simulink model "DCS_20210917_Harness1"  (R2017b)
settings: Solver=FixedStepDiscrete  StartTime=0.0  StopTime=10.0  FixedStep=0.01  RelTol=1e-3  EnableMultiTasking=on
undefined symbols (not defined in the file): sigbuilder_block
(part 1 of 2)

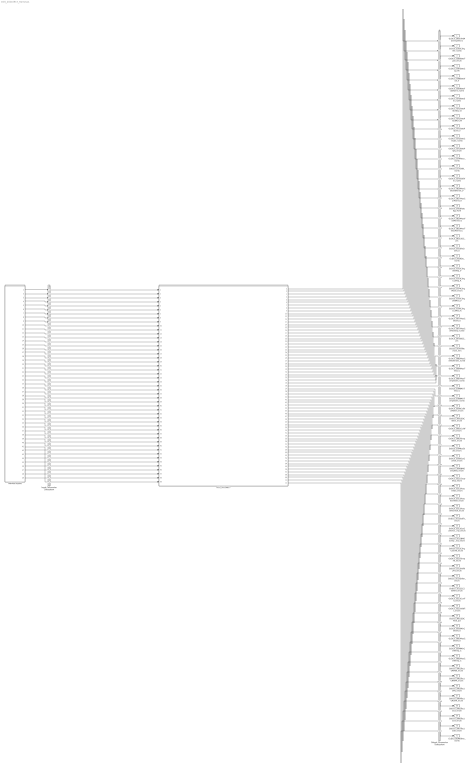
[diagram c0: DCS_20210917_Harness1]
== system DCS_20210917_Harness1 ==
  DCS_20210917 : ModelReference  ModelNameDialog=DCS_20210917  SimulationMode=Normal  ModelReferenceVersion='M106C105'
  Harness Inputs : Subsystem  Tag=STV Subsys  LoadFcn=sigbuilder_block('load');  StartFcn=sigbuilder_block('start');  StopFcn=sigbuilder_block('stop');  ClipboardFcn=sigbuilder_block('clipboard');  mask(Sigbuilder block){tuvar=[0:10]}
      mask init:
      | if ~strcmp(get_param(bdroot(gcb),'SimulationStatus'),'stopped'),tuvar = sigbuilder_block('maskInit'); end
  Input Conversion Subsystem : Subsystem  Tag=__SLT_ICS__  Description=Signal spec. and routing
  Output Conversion Subsystem : Subsystem  Tag=__SLT_OCS__  Description=Signal spec. and routing
  GcDCS_2601AlwMaxChrgVolt_V : Outport  OutDataTypeStr=fixdt('ufix16_Sp1')  PortDimensions=[1]
  GcDCS_2565ChrgVer_numb : Outport  Port=2  OutDataTypeStr=uint32  PortDimensions=[1]
  GeDCS_2566BattType_enum : Outport  Port=3  OutDataTypeStr=uint8  PortDimensions=[1]
  GcDCS_2567BattCap_Ah : Outport  Port=4  OutDataTypeStr=fixdt('ufix16_Sp1')  PortDimensions=[1]
  GcDCS_2568BattVolt_V : Outport  Port=5  OutDataTypeStr=fixdt('ufix16_Sp1')  PortDimensions=[1]
  GaDCS_2569BattFctyName_numb : Outport  Port=6  OutDataTypeStr=uint8  PortDimensions=[4]
  GcDCS_2570BattSer_numb : Outport  Port=7  OutDataTypeStr=uint32  PortDimensions=[1]
  GcDCS_2571BattPrdctDay_D : Outport  Port=8  OutDataTypeStr=uint8  PortDimensions=[1]
  GcDCS_2571BattPrdctMon_M : Outport  Port=9  OutDataTypeStr=uint8  PortDimensions=[1]
  GcDCS_2571BattPrdctYr_Y : Outport  Port=10  OutDataTypeStr=fixdt('ufix8_B1985')  PortDimensions=[1]
  GcDCS_2572BattChrgCt_numb : Outport  Port=11  OutDataTypeStr=uint32  PortDimensions=[1]
  GeDCS_2573BattPrpty_enum : Outport  Port=12  OutDataTypeStr=uint8  PortDimensions=[1]
  GcDCS_2574Resv_numb : Outport  Port=13  OutDataTypeStr=uint8  PortDimensions=[1]
  GaDCS_2575VIN_numb : Outport  Port=14  OutDataTypeStr=uint8  PortDimensions=[17]
  GaDCS_2576SoftVer_numb : Outport  Port=15  OutDataTypeStr=uint8  PortDimensions=[8]
  GcDCS_2816MaxCellVoltPermit_V : Outport  Port=16  OutDataTypeStr=single  PortDimensions=[1]
  GcDCS_2817MaxCurPermit_A : Outport  Port=17  OutDataTypeStr=fixdt('ufix16_Sp1_Bn400')  PortDimensions=[1]
  GcDCS_2818RateEgy_Kwh : Outport  Port=18  OutDataTypeStr=fixdt('ufix16_Sp1')  PortDimensions=[1]
  GcDCS_2819MaxVoltPermit_V : Outport  Port=19  OutDataTypeStr=fixdt('ufix16_Sp1')  PortDimensions=[1]
  GcDCS_2820MaxTempPermit_C : Outport  Port=20  OutDataTypeStr=fixdt('ufix8_Bn50')  PortDimensions=[1]
  GcDCS_2821SOC_pct : Outport  Port=21  OutDataTypeStr=fixdt('ufix16_Sp1')  PortDimensions=[1]
  GcDCS_2822PackVolt_V : Outport  Port=22  OutDataTypeStr=fixdt('ufix16_Sp1')  PortDimensions=[1]
  GcDCS_2829Da_numb : Outport  Port=23  OutDataTypeStr=uint8  PortDimensions=[1]
  GcDCS_3072ChrgVoltReq_V : Outport  Port=24  OutDataTypeStr=fixdt('ufix16_Sp1')  PortDimensions=[1]
  GcDCS_3073ChrgCurReq_A : Outport  Port=25  OutDataTypeStr=fixdt('ufix16_Sp1_Bn400')  PortDimensions=[1]
  GeDCS_3074ChrgMode_enum : Outport  Port=26  OutDataTypeStr=uint8  PortDimensions=[1]
  GcDCS_3075ChrgVoltMea_V : Outport  Port=27  OutDataTypeStr=fixdt('ufix16_Sp1')  PortDimensions=[1]
  GcDCS_3076ChrgCurMea_A : Outport  Port=28  OutDataTypeStr=fixdt('ufix16_Sp1_Bn400')  PortDimensions=[1]
  GcDCS_3077MaxCellVolt_V : Outport  Port=29  OutDataTypeStr=fixdt('ufix16_Sp01')  PortDimensions=[1]
  GcDCS_3077MaxCellVoltGrp_numb : Outport  Port=30  OutDataTypeStr=uint8  PortDimensions=[1]
  GcDCS_3078SOC_pct : Outport  Port=31  OutDataTypeStr=uint8  PortDimensions=[1]
  GcDCS_3079TiRemain_min : Outport  Port=32  OutDataTypeStr=uint16  PortDimensions=[1]
  GcDCS_3085MaxCellVoltIndex_numb : Outport  Port=33  OutDataTypeStr=fixdt('ufix8_B1')  PortDimensions=[1]
  GcDCS_3086MaxTemp_C : Outport  Port=34  OutDataTypeStr=fixdt('ufix8_Bn50')  PortDimensions=[1]
  GcDCS_3087MaxTempIndex_numb : Outport  Port=35  OutDataTypeStr=fixdt('ufix8_B1')  PortDimensions=[1]
  GcDCS_3088MinTemp_C : Outport  Port=36  OutDataTypeStr=fixdt('ufix8_Bn50')  PortDimensions=[1]
  GcDCS_3089MinTempIndex_numb : Outport  Port=37  OutDataTypeStr=fixdt('ufix8_B1')  PortDimensions=[1]
  GeDCS_3090CellVoltWarn_enum : Outport  Port=38  OutDataTypeStr=uint8  PortDimensions=[1]
  GeDCS_3091SOCWarn_enum : Outport  Port=39  OutDataTypeStr=uint8  PortDimensions=[1]
  GeDCS_3092CurWarn_enum : Outport  Port=40  OutDataTypeStr=uint8  PortDimensions=[1]
  GeDCS_3093TempWarn_enum : Outport  Port=41  OutDataTypeStr=uint8  PortDimensions=[1]
  GeDCS_3094IsoState_enum : Outport  Port=42  OutDataTypeStr=uint8  PortDimensions=[1]
  GeDCS_3095OutContSt_enum : Outport  Port=43  OutDataTypeStr=uint8  PortDimensions=[1]
  GeDCS_3096BMSChrgRdy_enum : Outport  Port=44  OutDataTypeStr=uint8  PortDimensions=[1]
  GeDCS_3511ChrgrStop_enum : Outport  Port=45  OutDataTypeStr=uint8  PortDimensions=[1]
  GeDCS_3511ReachSOC_enum : Outport  Port=46  OutDataTypeStr=uint8  PortDimensions=[1]
  GeDCS_3511ReachCellVolt_enum : Outport  Port=47  OutDataTypeStr=uint8  PortDimensions=[1]
  GeDCS_3511ReachPackVolt_enum : Outport  Port=48  OutDataTypeStr=uint8  PortDimensions=[1]
  GeDCS_3512IsoFlt_enum : Outport  Port=49  OutDataTypeStr=uint8  PortDimensions=[1]
  GeDCS_3512OutContOverTemp_enum : Outport  Port=50  OutDataTypeStr=uint8  PortDimensions=[1]
  GeDCS_3512BMSCompOverTemp_enum : Outport  Port=51  OutDataTypeStr=uint8  PortDimensions=[1]
  GeDCS_3512ChrgContFlt_enum : Outport  Port=52  OutDataTypeStr=uint8  PortDimensions=[1]
  GeDCS_3512TempFlt_enum : Outport  Port=53  OutDataTypeStr=uint8  PortDimensions=[1]
  GeDCS_3512HVRlyFlt_enum : Outport  Port=54  OutDataTypeStr=uint8  PortDimensions=[1]
  GeDCS_3512Other_enum : Outport  Port=55  OutDataTypeStr=uint8  PortDimensions=[1]
  GeDCS_3512CC2VoltFlt_enum : Outport  Port=56  OutDataTypeStr=uint8  PortDimensions=[1]
  GeDCS_3513CurrFlt_enum : Outport  Port=57  OutDataTypeStr=uint8  PortDimensions=[1]
  GeDCS_3513VoltFlt_enum : Outport  Port=58  OutDataTypeStr=uint8  PortDimensions=[1]
  GcDCS_3601SOCFinal_pct : Outport  Port=59  OutDataTypeStr=uint8  PortDimensions=[1]
  GcDCS_3602MinCellVolt_V : Outport  Port=60  OutDataTypeStr=fixdt('ufix16_Sp01')  PortDimensions=[1]
  GcDCS_3603MaxCellVolt_V : Outport  Port=61  OutDataTypeStr=fixdt('ufix16_Sp01')  PortDimensions=[1]
  GcDCS_3604MinCellTemp_C : Outport  Port=62  OutDataTypeStr=fixdt('ufix8_Bn50')  PortDimensions=[1]
  GcDCS_3605MaxCellTemp_C : Outport  Port=63  OutDataTypeStr=fixdt('ufix8_Bn50')  PortDimensions=[1]
  GeDCS_3901ToutCRM00_enum : Outport  Port=64  OutDataTypeStr=uint8  PortDimensions=[1]
  GeDCS_3902ToutCRMAA_enum : Outport  Port=65  OutDataTypeStr=uint8  PortDimensions=[1]
  GeDCS_3903ToutCML_enum : Outport  Port=66  OutDataTypeStr=uint8  PortDimensions=[1]
  GeDCS_3904ToutCROAA_enum : Outport  Port=67  OutDataTypeStr=uint8  PortDimensions=[1]
  GeDCS_3905ToutCCS_enum : Outport  Port=68  OutDataTypeStr=uint8  PortDimensions=[1]
  GeDCS_3906ToutCST_enum : Outport  Port=69  OutDataTypeStr=uint8  PortDimensions=[1]
  GeDCS_3907ToutCSD_enum : Outport  Port=70  OutDataTypeStr=uint8  PortDimensions=[1]
  GcDCS_BEMOther_numb : Outport  Port=71  OutDataTypeStr=uint8  PortDimensions=[1]
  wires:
  Harness Inputs/1(GbDCC_BSTMsgCmd_flg) -> Input Conversion Subsystem/1(Inport_1)
  Harness Inputs/2(GcDCC_DCChrgVoltRqst_V) -> Input Conversion Subsystem/2(Inport_2)
  Harness Inputs/3(GbDCC_DCChrgVerSta_flg) -> Input Conversion Subsystem/3(Inport_3)
  Harness Inputs/4(GcDCC_DCChrgCrntRqst_A) -> Input Conversion Subsystem/4(Inport_4)
  Harness Inputs/5(GcHDP_PackCrnt_A) -> Input Conversion Subsystem/5(Inport_5)
  Harness Inputs/6(GcCDP_MaxCellVoltNumb_numb) -> Input Conversion Subsystem/6(Inport_6)
  Harness Inputs/7(GcSOC_DispSOC_pct) -> Input Conversion Subsystem/7(Inport_7)
  Harness Inputs/8(GcDCC_ChrgingTiRem_min) -> Input Conversion Subsystem/8(Inport_8)
  Harness Inputs/9(GcCDP_MaxCellTemp_C) -> Input Conversion Subsystem/9(Inport_9)
  Harness Inputs/10(GcCDP_MaxCellTempNumb_numb) -> Input Conversion Subsystem/10(Inport_10)
  Harness Inputs/11(GcCDP_MinCellTemp_C) -> Input Conversion Subsystem/11(Inport_11)
  Harness Inputs/12(GcCDP_MinCellTempNumb_numb) -> Input Conversion Subsystem/12(Inport_12)
  Harness Inputs/13(GbDCC_DCChrgFinish_flg) -> Input Conversion Subsystem/13(Inport_13)
  Harness Inputs/14(GeISO_ResFltLvl_enum) -> Input Conversion Subsystem/14(Inport_14)
  Harness Inputs/15(GeLDP_DCPlugTempState_enum) -> Input Conversion Subsystem/15(Inport_15)
  Harness Inputs/16(GbISP_TFCellTempHiFltLv2_flg) -> Input Conversion Subsystem/16(Inport_16)
  Harness Inputs/17(GbCTD_DCPosCloseFlt_flg) -> Input Conversion Subsystem/17(Inport_17)
  Harness Inputs/18(GbCTD_DCPosOpenFlt_flg) -> Input Conversion Subsystem/18(Inport_18)
  Harness Inputs/19(GeFTC_FltLevel_enum) -> Input Conversion Subsystem/19(Inport_19)
  Harness Inputs/20(GeSOP_ChrgPwrState_enum) -> Input Conversion Subsystem/20(Inport_20)
  Harness Inputs/21(GbISP_TFCellVoltHiFltLv2_flg) -> Input Conversion Subsystem/21(Inport_21)
  Harness Inputs/22(GcCDP_MinCellVolt_mV) -> Input Conversion Subsystem/22(Inport_22)
  Harness Inputs/23(GcCDP_MaxCellVolt_mV) -> Input Conversion Subsystem/23(Inport_23)
  Harness Inputs/24(GbDCC_CRM00Tout_flg) -> Input Conversion Subsystem/24(Inport_24)
  Harness Inputs/25(GbDCC_CRMAATout_flg) -> Input Conversion Subsystem/25(Inport_25)
  Harness Inputs/26(GbDCC_CMLTout_flg) -> Input Conversion Subsystem/26(Inport_26)
  Harness Inputs/27(GbDCC_CROAATout_flg) -> Input Conversion Subsystem/27(Inport_27)
  Harness Inputs/28(GbDCC_CCSTout_flg) -> Input Conversion Subsystem/28(Inport_28)
  Harness Inputs/29(GbDCC_CSTTout_flg) -> Input Conversion Subsystem/29(Inport_29)
  Harness Inputs/30(GbDCC_CSDTout_flg) -> Input Conversion Subsystem/30(Inport_30)
  Harness Inputs/31(GbGDP_CSTRecOnce_flg) -> Input Conversion Subsystem/31(Inport_31)
  Harness Inputs/32(GcHDP_PackVolt_V) -> Input Conversion Subsystem/32(Inport_32)
  Harness Inputs/33(GeCTC_CtrCtlState_enum) -> Input Conversion Subsystem/33(Inport_33)
  Harness Inputs/34(GbDCC_CROTout_flg) -> Input Conversion Subsystem/34(Inport_34)
  Harness Inputs/35(GbDCC_DCCrntUnctrolFlt_flg) -> Input Conversion Subsystem/35(Inport_35)
  Harness Inputs/36(GbLDP_CC2STG_flg) -> Input Conversion Subsystem/36(Inport_36)
  Harness Inputs/37(GbLDP_CC2VoltRaty_flg) -> Input Conversion Subsystem/37(Inport_37)
  Harness Inputs/38(GcADP_VinCode1_numb) -> Input Conversion Subsystem/38(Inport_38)
  Harness Inputs/39(GcADP_VinCode2_numb) -> Input Conversion Subsystem/39(Inport_39)
  Harness Inputs/40(GcADP_VinCode3_numb) -> Input Conversion Subsystem/40(Inport_40)
  Harness Inputs/41(GcADP_VinCode4_numb) -> Input Conversion Subsystem/41(Inport_41)
  Harness Inputs/42(GcADP_VinCode5_numb) -> Input Conversion Subsystem/42(Inport_42)
  Harness Inputs/43(GcADP_VinCode6_numb) -> Input Conversion Subsystem/43(Inport_43)
  Harness Inputs/44(GcADP_VinCode7_numb) -> Input Conversion Subsystem/44(Inport_44)
  Harness Inputs/45(GcADP_VinCodeNum_numb) -> Input Conversion Subsystem/45(Inport_45)
  Harness Inputs/46(GeCTC_CtrCtlConnMode_enum) -> Input Conversion Subsystem/46(Inport_46)
  Harness Inputs/47(GcUDS_FullChrgCutoffVolt_mV) -> Input Conversion Subsystem/47(Inport_47)
  Harness Inputs/48(GcUDS_BatEnergy_kWh) -> Input Conversion Subsystem/48(Inport_48)
  Harness Inputs/49(GeUDS_CapSel_enum) -> Input Conversion Subsystem/49(Inport_49)
  Output Conversion Subsystem/1(Outport_1) -> GcDCS_2601AlwMaxChrgVolt_V/1
  Output Conversion Subsystem/2(Outport_2) -> GcDCS_2565ChrgVer_numb/1
  Output Conversion Subsystem/3(Outport_3) -> GeDCS_2566BattType_enum/1
  Output Conversion Subsystem/4(Outport_4) -> GcDCS_2567BattCap_Ah/1
  Output Conversion Subsystem/5(Outport_5) -> GcDCS_2568BattVolt_V/1
  Output Conversion Subsystem/6(Outport_6) -> GaDCS_2569BattFctyName_numb/1
  Output Conversion Subsystem/7(Outport_7) -> GcDCS_2570BattSer_numb/1
  Output Conversion Subsystem/8(Outport_8) -> GcDCS_2571BattPrdctDay_D/1
  Output Conversion Subsystem/9(Outport_9) -> GcDCS_2571BattPrdctMon_M/1
  Output Conversion Subsystem/10(Outport_10) -> GcDCS_2571BattPrdctYr_Y/1
  Output Conversion Subsystem/11(Outport_11) -> GcDCS_2572BattChrgCt_numb/1
  Output Conversion Subsystem/12(Outport_12) -> GeDCS_2573BattPrpty_enum/1
  Output Conversion Subsystem/13(Outport_13) -> GcDCS_2574Resv_numb/1
  Output Conversion Subsystem/14(Outport_14) -> GaDCS_2575VIN_numb/1
  Output Conversion Subsystem/15(Outport_15) -> GaDCS_2576SoftVer_numb/1
  Output Conversion Subsystem/16(Outport_16) -> GcDCS_2816MaxCellVoltPermit_V/1
  Output Conversion Subsystem/17(Outport_17) -> GcDCS_2817MaxCurPermit_A/1
  Output Conversion Subsystem/18(Outport_18) -> GcDCS_2818RateEgy_Kwh/1
  Output Conversion Subsystem/19(Outport_19) -> GcDCS_2819MaxVoltPermit_V/1
  Output Conversion Subsystem/20(Outport_20) -> GcDCS_2820MaxTempPermit_C/1
  Output Conversion Subsystem/21(Outport_21) -> GcDCS_2821SOC_pct/1
  Output Conversion Subsystem/22(Outport_22) -> GcDCS_2822PackVolt_V/1
  Output Conversion Subsystem/23(Outport_23) -> GcDCS_2829Da_numb/1
  Output Conversion Subsystem/24(Outport_24) -> GcDCS_3072ChrgVoltReq_V/1
  Output Conversion Subsystem/25(Outport_25) -> GcDCS_3073ChrgCurReq_A/1
  Output Conversion Subsystem/26(Outport_26) -> GeDCS_3074ChrgMode_enum/1
  Output Conversion Subsystem/27(Outport_27) -> GcDCS_3075ChrgVoltMea_V/1
  Output Conversion Subsystem/28(Outport_28) -> GcDCS_3076ChrgCurMea_A/1
  Output Conversion Subsystem/29(Outport_29) -> GcDCS_3077MaxCellVolt_V/1
  Output Conversion Subsystem/30(Outport_30) -> GcDCS_3077MaxCellVoltGrp_numb/1
  Output Conversion Subsystem/31(Outport_31) -> GcDCS_3078SOC_pct/1
  Output Conversion Subsystem/32(Outport_32) -> GcDCS_3079TiRemain_min/1
  Output Conversion Subsystem/33(Outport_33) -> GcDCS_3085MaxCellVoltIndex_numb/1
  Output Conversion Subsystem/34(Outport_34) -> GcDCS_3086MaxTemp_C/1
  Output Conversion Subsystem/35(Outport_35) -> GcDCS_3087MaxTempIndex_numb/1
  Output Conversion Subsystem/36(Outport_36) -> GcDCS_3088MinTemp_C/1
  Output Conversion Subsystem/37(Outport_37) -> GcDCS_3089MinTempIndex_numb/1
  Output Conversion Subsystem/38(Outport_38) -> GeDCS_3090CellVoltWarn_enum/1
  Output Conversion Subsystem/39(Outport_39) -> GeDCS_3091SOCWarn_enum/1
  Output Conversion Subsystem/40(Outport_40) -> GeDCS_3092CurWarn_enum/1
  Output Conversion Subsystem/41(Outport_41) -> GeDCS_3093TempWarn_enum/1
  Output Conversion Subsystem/42(Outport_42) -> GeDCS_3094IsoState_enum/1
  Output Conversion Subsystem/43(Outport_43) -> GeDCS_3095OutContSt_enum/1
  Output Conversion Subsystem/44(Outport_44) -> GeDCS_3096BMSChrgRdy_enum/1
  Output Conversion Subsystem/45(Outport_45) -> GeDCS_3511ChrgrStop_enum/1
  Output Conversion Subsystem/46(Outport_46) -> GeDCS_3511ReachSOC_enum/1
  Output Conversion Subsystem/47(Outport_47) -> GeDCS_3511ReachCellVolt_enum/1
  Output Conversion Subsystem/48(Outport_48) -> GeDCS_3511ReachPackVolt_enum/1
  Output Conversion Subsystem/49(Outport_49) -> GeDCS_3512IsoFlt_enum/1
  Output Conversion Subsystem/50(Outport_50) -> GeDCS_3512OutContOverTemp_enum/1
  Output Conversion Subsystem/51(Outport_51) -> GeDCS_3512BMSCompOverTemp_enum/1
  Output Conversion Subsystem/52(Outport_52) -> GeDCS_3512ChrgContFlt_enum/1
  Output Conversion Subsystem/53(Outport_53) -> GeDCS_3512TempFlt_enum/1
  Output Conversion Subsystem/54(Outport_54) -> GeDCS_3512HVRlyFlt_enum/1
  Output Conversion Subsystem/55(Outport_55) -> GeDCS_3512Other_enum/1
  Output Conversion Subsystem/56(Outport_56) -> GeDCS_3512CC2VoltFlt_enum/1
  Output Conversion Subsystem/57(Outport_57) -> GeDCS_3513CurrFlt_enum/1
  Output Conversion Subsystem/58(Outport_58) -> GeDCS_3513VoltFlt_enum/1
  Output Conversion Subsystem/59(Outport_59) -> GcDCS_3601SOCFinal_pct/1
  Output Conversion Subsystem/60(Outport_60) -> GcDCS_3602MinCellVolt_V/1
  Output Conversion Subsystem/61(Outport_61) -> GcDCS_3603MaxCellVolt_V/1
  Output Conversion Subsystem/62(Outport_62) -> GcDCS_3604MinCellTemp_C/1
  Output Conversion Subsystem/63(Outport_63) -> GcDCS_3605MaxCellTemp_C/1
  Output Conversion Subsystem/64(Outport_64) -> GeDCS_3901ToutCRM00_enum/1
  Output Conversion Subsystem/65(Outport_65) -> GeDCS_3902ToutCRMAA_enum/1
  Output Conversion Subsystem/66(Outport_66) -> GeDCS_3903ToutCML_enum/1
  Output Conversion Subsystem/67(Outport_67) -> GeDCS_3904ToutCROAA_enum/1
  Output Conversion Subsystem/68(Outport_68) -> GeDCS_3905ToutCCS_enum/1
  Output Conversion Subsystem/69(Outport_69) -> GeDCS_3906ToutCST_enum/1
  Output Conversion Subsystem/70(Outport_70) -> GeDCS_3907ToutCSD_enum/1
  Output Conversion Subsystem/71(Outport_71) -> GcDCS_BEMOther_numb/1
  Input Conversion Subsystem/1(Outport_1) -> DCS_20210917/1
  Input Conversion Subsystem/2(Outport_2) -> DCS_20210917/2
  Input Conversion Subsystem/3(Outport_3) -> DCS_20210917/3
  Input Conversion Subsystem/4(Outport_4) -> DCS_20210917/4
  Input Conversion Subsystem/5(Outport_5) -> DCS_20210917/5
  Input Conversion Subsystem/6(Outport_6) -> DCS_20210917/6
  Input Conversion Subsystem/7(Outport_7) -> DCS_20210917/7
  Input Conversion Subsystem/8(Outport_8) -> DCS_20210917/8
  Input Conversion Subsystem/9(Outport_9) -> DCS_20210917/9
  Input Conversion Subsystem/10(Outport_10) -> DCS_20210917/10
  Input Conversion Subsystem/11(Outport_11) -> DCS_20210917/11
  Input Conversion Subsystem/12(Outport_12) -> DCS_20210917/12
  Input Conversion Subsystem/13(Outport_13) -> DCS_20210917/13
  Input Conversion Subsystem/14(Outport_14) -> DCS_20210917/14
  Input Conversion Subsystem/15(Outport_15) -> DCS_20210917/15
  Input Conversion Subsystem/16(Outport_16) -> DCS_20210917/16
  Input Conversion Subsystem/17(Outport_17) -> DCS_20210917/17
  Input Conversion Subsystem/18(Outport_18) -> DCS_20210917/18
  Input Conversion Subsystem/19(Outport_19) -> DCS_20210917/19
  Input Conversion Subsystem/20(Outport_20) -> DCS_20210917/20
  Input Conversion Subsystem/21(Outport_21) -> DCS_20210917/21
  Input Conversion Subsystem/22(Outport_22) -> DCS_20210917/22
  Input Conversion Subsystem/23(Outport_23) -> DCS_20210917/23
  Input Conversion Subsystem/24(Outport_24) -> DCS_20210917/24
  Input Conversion Subsystem/25(Outport_25) -> DCS_20210917/25
  Input Conversion Subsystem/26(Outport_26) -> DCS_20210917/26
  Input Conversion Subsystem/27(Outport_27) -> DCS_20210917/27
  Input Conversion Subsystem/28(Outport_28) -> DCS_20210917/28
  Input Conversion Subsystem/29(Outport_29) -> DCS_20210917/29
  Input Conversion Subsystem/30(Outport_30) -> DCS_20210917/30
  Input Conversion Subsystem/31(Outport_31) -> DCS_20210917/31
  Input Conversion Subsystem/32(Outport_32) -> DCS_20210917/32
  Input Conversion Subsystem/33(Outport_33) -> DCS_20210917/33
  Input Conversion Subsystem/34(Outport_34) -> DCS_20210917/34
  Input Conversion Subsystem/35(Outport_35) -> DCS_20210917/35
  Input Conversion Subsystem/36(Outport_36) -> DCS_20210917/36
  Input Conversion Subsystem/37(Outport_37) -> DCS_20210917/37
  Input Conversion Subsystem/38(Outport_38) -> DCS_20210917/38
  Input Conversion Subsystem/39(Outport_39) -> DCS_20210917/39
  Input Conversion Subsystem/40(Outport_40) -> DCS_20210917/40
  Input Conversion Subsystem/41(Outport_41) -> DCS_20210917/41
  Input Conversion Subsystem/42(Outport_42) -> DCS_20210917/42
  Input Conversion Subsystem/43(Outport_43) -> DCS_20210917/43
  Input Conversion Subsystem/44(Outport_44) -> DCS_20210917/44
  Input Conversion Subsystem/45(Outport_45) -> DCS_20210917/45
  Input Conversion Subsystem/46(Outport_46) -> DCS_20210917/46
  Input Conversion Subsystem/47(Outport_47) -> DCS_20210917/47
  Input Conversion Subsystem/48(Outport_48) -> DCS_20210917/48
  Input Conversion Subsystem/49(Outport_49) -> DCS_20210917/49
  DCS_20210917/1 -> Output Conversion Subsystem/1(Inport_1)
  DCS_20210917/2 -> Output Conversion Subsystem/2(Inport_2)
  DCS_20210917/3 -> Output Conversion Subsystem/3(Inport_3)
  DCS_20210917/4 -> Output Conversion Subsystem/4(Inport_4)
  DCS_20210917/5 -> Output Conversion Subsystem/5(Inport_5)
  DCS_20210917/6 -> Output Conversion Subsystem/6(Inport_6)
  DCS_20210917/7 -> Output Conversion Subsystem/7(Inport_7)
  DCS_20210917/8 -> Output Conversion Subsystem/8(Inport_8)
  DCS_20210917/9 -> Output Conversion Subsystem/9(Inport_9)
  DCS_20210917/10 -> Output Conversion Subsystem/10(Inport_10)
  DCS_20210917/11 -> Output Conversion Subsystem/11(Inport_11)
  DCS_20210917/12 -> Output Conversion Subsystem/12(Inport_12)
  DCS_20210917/13 -> Output Conversion Subsystem/13(Inport_13)
  DCS_20210917/14 -> Output Conversion Subsystem/14(Inport_14)
  DCS_20210917/15 -> Output Conversion Subsystem/15(Inport_15)
  DCS_20210917/16 -> Output Conversion Subsystem/16(Inport_16)
  DCS_20210917/17 -> Output Conversion Subsystem/17(Inport_17)
  DCS_20210917/18 -> Output Conversion Subsystem/18(Inport_18)
  DCS_20210917/19 -> Output Conversion Subsystem/19(Inport_19)
  DCS_20210917/20 -> Output Conversion Subsystem/20(Inport_20)
  DCS_20210917/21 -> Output Conversion Subsystem/21(Inport_21)
  DCS_20210917/22 -> Output Conversion Subsystem/22(Inport_22)
  DCS_20210917/23 -> Output Conversion Subsystem/23(Inport_23)
  DCS_20210917/24 -> Output Conversion Subsystem/24(Inport_24)
  DCS_20210917/25 -> Output Conversion Subsystem/25(Inport_25)
  DCS_20210917/26 -> Output Conversion Subsystem/26(Inport_26)
  DCS_20210917/27 -> Output Conversion Subsystem/27(Inport_27)
  DCS_20210917/28 -> Output Conversion Subsystem/28(Inport_28)
  DCS_20210917/29 -> Output Conversion Subsystem/29(Inport_29)
  DCS_20210917/30 -> Output Conversion Subsystem/30(Inport_30)
  DCS_20210917/31 -> Output Conversion Subsystem/31(Inport_31)
  DCS_20210917/32 -> Output Conversion Subsystem/32(Inport_32)
  DCS_20210917/33 -> Output Conversion Subsystem/33(Inport_33)
  DCS_20210917/34 -> Output Conversion Subsystem/34(Inport_34)
  DCS_20210917/35 -> Output Conversion Subsystem/35(Inport_35)
  DCS_20210917/36 -> Output Conversion Subsystem/36(Inport_36)
  DCS_20210917/37 -> Output Conversion Subsystem/37(Inport_37)
  DCS_20210917/38 -> Output Conversion Subsystem/38(Inport_38)
  DCS_20210917/39 -> Output Conversion Subsystem/39(Inport_39)
  DCS_20210917/40 -> Output Conversion Subsystem/40(Inport_40)
  DCS_20210917/41 -> Output Conversion Subsystem/41(Inport_41)
  DCS_20210917/42 -> Output Conversion Subsystem/42(Inport_42)
  DCS_20210917/43 -> Output Conversion Subsystem/43(Inport_43)
  DCS_20210917/44 -> Output Conversion Subsystem/44(Inport_44)
  DCS_20210917/45 -> Output Conversion Subsystem/45(Inport_45)
  DCS_20210917/46 -> Output Conversion Subsystem/46(Inport_46)
  DCS_20210917/47 -> Output Conversion Subsystem/47(Inport_47)
  DCS_20210917/48 -> Output Conversion Subsystem/48(Inport_48)
  DCS_20210917/49 -> Output Conversion Subsystem/49(Inport_49)
  DCS_20210917/50 -> Output Conversion Subsystem/50(Inport_50)
  DCS_20210917/51 -> Output Conversion Subsystem/51(Inport_51)
  DCS_20210917/52 -> Output Conversion Subsystem/52(Inport_52)
  DCS_20210917/53 -> Output Conversion Subsystem/53(Inport_53)
  DCS_20210917/54 -> Output Conversion Subsystem/54(Inport_54)
  DCS_20210917/55 -> Output Conversion Subsystem/55(Inport_55)
  DCS_20210917/56 -> Output Conversion Subsystem/56(Inport_56)
  DCS_20210917/57 -> Output Conversion Subsystem/57(Inport_57)
  DCS_20210917/58 -> Output Conversion Subsystem/58(Inport_58)
  DCS_20210917/59 -> Output Conversion Subsystem/59(Inport_59)
  DCS_20210917/60 -> Output Conversion Subsystem/60(Inport_60)
  DCS_20210917/61 -> Output Conversion Subsystem/61(Inport_61)
  DCS_20210917/62 -> Output Conversion Subsystem/62(Inport_62)
  DCS_20210917/63 -> Output Conversion Subsystem/63(Inport_63)
  DCS_20210917/64 -> Output Conversion Subsystem/64(Inport_64)
  DCS_20210917/65 -> Output Conversion Subsystem/65(Inport_65)
  DCS_20210917/66 -> Output Conversion Subsystem/66(Inport_66)
  DCS_20210917/67 -> Output Conversion Subsystem/67(Inport_67)
  DCS_20210917/68 -> Output Conversion Subsystem/68(Inport_68)
  DCS_20210917/69 -> Output Conversion Subsystem/69(Inport_69)
  DCS_20210917/70 -> Output Conversion Subsystem/70(Inport_70)
  DCS_20210917/71 -> Output Conversion Subsystem/71(Inport_71)

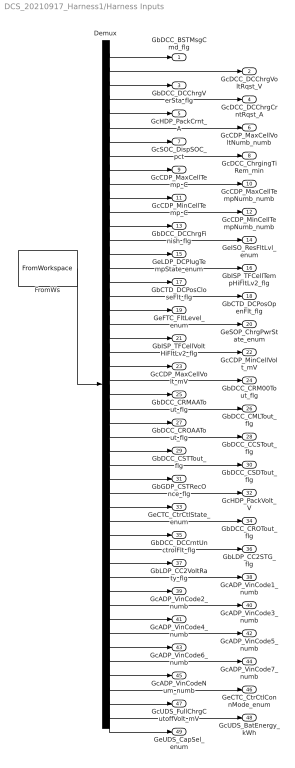
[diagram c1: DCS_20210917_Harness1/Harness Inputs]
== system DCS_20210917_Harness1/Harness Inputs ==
  Demux : Demux  Tag=STV Demux  Outputs=49
  FromWs : FromWorkspace  Tag=STV FromWs  VariableName=tuvar  SampleTime=0
  GbDCC_BSTMsgCmd_flg : Outport  Tag=STV Outport
  GcDCC_DCChrgVoltRqst_V : Outport  Tag=STV Outport  Port=2
  GbDCC_DCChrgVerSta_flg : Outport  Tag=STV Outport  Port=3
  GcDCC_DCChrgCrntRqst_A : Outport  Tag=STV Outport  Port=4
  GcHDP_PackCrnt_A : Outport  Tag=STV Outport  Port=5
  GcCDP_MaxCellVoltNumb_numb : Outport  Tag=STV Outport  Port=6
  GcSOC_DispSOC_pct : Outport  Tag=STV Outport  Port=7
  GcDCC_ChrgingTiRem_min : Outport  Tag=STV Outport  Port=8
  GcCDP_MaxCellTemp_C : Outport  Tag=STV Outport  Port=9
  GcCDP_MaxCellTempNumb_numb : Outport  Tag=STV Outport  Port=10
  GcCDP_MinCellTemp_C : Outport  Tag=STV Outport  Port=11
  GcCDP_MinCellTempNumb_numb : Outport  Tag=STV Outport  Port=12
  GbDCC_DCChrgFinish_flg : Outport  Tag=STV Outport  Port=13
  GeISO_ResFltLvl_enum : Outport  Tag=STV Outport  Port=14
  GeLDP_DCPlugTempState_enum : Outport  Tag=STV Outport  Port=15
  GbISP_TFCellTempHiFltLv2_flg : Outport  Tag=STV Outport  Port=16
  GbCTD_DCPosCloseFlt_flg : Outport  Tag=STV Outport  Port=17
  GbCTD_DCPosOpenFlt_flg : Outport  Tag=STV Outport  Port=18
  GeFTC_FltLevel_enum : Outport  Tag=STV Outport  Port=19
  GeSOP_ChrgPwrState_enum : Outport  Tag=STV Outport  Port=20
  GbISP_TFCellVoltHiFltLv2_flg : Outport  Tag=STV Outport  Port=21
  GcCDP_MinCellVolt_mV : Outport  Tag=STV Outport  Port=22
  GcCDP_MaxCellVolt_mV : Outport  Tag=STV Outport  Port=23
  GbDCC_CRM00Tout_flg : Outport  Tag=STV Outport  Port=24
  GbDCC_CRMAATout_flg : Outport  Tag=STV Outport  Port=25
  GbDCC_CMLTout_flg : Outport  Tag=STV Outport  Port=26
  GbDCC_CROAATout_flg : Outport  Tag=STV Outport  Port=27
  GbDCC_CCSTout_flg : Outport  Tag=STV Outport  Port=28
  GbDCC_CSTTout_flg : Outport  Tag=STV Outport  Port=29
  GbDCC_CSDTout_flg : Outport  Tag=STV Outport  Port=30
  GbGDP_CSTRecOnce_flg : Outport  Tag=STV Outport  Port=31
  GcHDP_PackVolt_V : Outport  Tag=STV Outport  Port=32
  GeCTC_CtrCtlState_enum : Outport  Tag=STV Outport  Port=33
  GbDCC_CROTout_flg : Outport  Tag=STV Outport  Port=34
  GbDCC_DCCrntUnctrolFlt_flg : Outport  Tag=STV Outport  Port=35
  GbLDP_CC2STG_flg : Outport  Tag=STV Outport  Port=36
  GbLDP_CC2VoltRaty_flg : Outport  Tag=STV Outport  Port=37
  GcADP_VinCode1_numb : Outport  Tag=STV Outport  Port=38
  GcADP_VinCode2_numb : Outport  Tag=STV Outport  Port=39
  GcADP_VinCode3_numb : Outport  Tag=STV Outport  Port=40
  GcADP_VinCode4_numb : Outport  Tag=STV Outport  Port=41
  GcADP_VinCode5_numb : Outport  Tag=STV Outport  Port=42
  GcADP_VinCode6_numb : Outport  Tag=STV Outport  Port=43
  GcADP_VinCode7_numb : Outport  Tag=STV Outport  Port=44
  GcADP_VinCodeNum_numb : Outport  Tag=STV Outport  Port=45
  GeCTC_CtrCtlConnMode_enum : Outport  Tag=STV Outport  Port=46
  GcUDS_FullChrgCutoffVolt_mV : Outport  Tag=STV Outport  Port=47
  GcUDS_BatEnergy_kWh : Outport  Tag=STV Outport  Port=48
  GeUDS_CapSel_enum : Outport  Tag=STV Outport  Port=49
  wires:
  FromWs/1 -> Demux/1
  Demux/1 -> GbDCC_BSTMsgCmd_flg/1
  Demux/2 -> GcDCC_DCChrgVoltRqst_V/1
  Demux/3 -> GbDCC_DCChrgVerSta_flg/1
  Demux/4 -> GcDCC_DCChrgCrntRqst_A/1
  Demux/5 -> GcHDP_PackCrnt_A/1
  Demux/6 -> GcCDP_MaxCellVoltNumb_numb/1
  Demux/7 -> GcSOC_DispSOC_pct/1
  Demux/8 -> GcDCC_ChrgingTiRem_min/1
  Demux/9 -> GcCDP_MaxCellTemp_C/1
  Demux/10 -> GcCDP_MaxCellTempNumb_numb/1
  Demux/11 -> GcCDP_MinCellTemp_C/1
  Demux/12 -> GcCDP_MinCellTempNumb_numb/1
  Demux/13 -> GbDCC_DCChrgFinish_flg/1
  Demux/14 -> GeISO_ResFltLvl_enum/1
  Demux/15 -> GeLDP_DCPlugTempState_enum/1
  Demux/16 -> GbISP_TFCellTempHiFltLv2_flg/1
  Demux/17 -> GbCTD_DCPosCloseFlt_flg/1
  Demux/18 -> GbCTD_DCPosOpenFlt_flg/1
  Demux/19 -> GeFTC_FltLevel_enum/1
  Demux/20 -> GeSOP_ChrgPwrState_enum/1
  Demux/21 -> GbISP_TFCellVoltHiFltLv2_flg/1
  Demux/22 -> GcCDP_MinCellVolt_mV/1
  Demux/23 -> GcCDP_MaxCellVolt_mV/1
  Demux/24 -> GbDCC_CRM00Tout_flg/1
  Demux/25 -> GbDCC_CRMAATout_flg/1
  Demux/26 -> GbDCC_CMLTout_flg/1
  Demux/27 -> GbDCC_CROAATout_flg/1
  Demux/28 -> GbDCC_CCSTout_flg/1
  Demux/29 -> GbDCC_CSTTout_flg/1
  Demux/30 -> GbDCC_CSDTout_flg/1
  Demux/31 -> GbGDP_CSTRecOnce_flg/1
  Demux/32 -> GcHDP_PackVolt_V/1
  Demux/33 -> GeCTC_CtrCtlState_enum/1
  Demux/34 -> GbDCC_CROTout_flg/1
  Demux/35 -> GbDCC_DCCrntUnctrolFlt_flg/1
  Demux/36 -> GbLDP_CC2STG_flg/1
  Demux/37 -> GbLDP_CC2VoltRaty_flg/1
  Demux/38 -> GcADP_VinCode1_numb/1
  Demux/39 -> GcADP_VinCode2_numb/1
  Demux/40 -> GcADP_VinCode3_numb/1
  Demux/41 -> GcADP_VinCode4_numb/1
  Demux/42 -> GcADP_VinCode5_numb/1
  Demux/43 -> GcADP_VinCode6_numb/1
  Demux/44 -> GcADP_VinCode7_numb/1
  Demux/45 -> GcADP_VinCodeNum_numb/1
  Demux/46 -> GeCTC_CtrCtlConnMode_enum/1
  Demux/47 -> GcUDS_FullChrgCutoffVolt_mV/1
  Demux/48 -> GcUDS_BatEnergy_kWh/1
  Demux/49 -> GeUDS_CapSel_enum/1

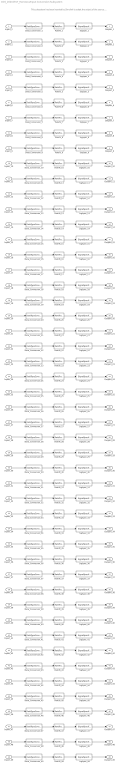
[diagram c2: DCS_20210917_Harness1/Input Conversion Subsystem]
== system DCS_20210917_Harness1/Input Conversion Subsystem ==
  note: This subsystem has been inserted by Simulink to adapt the output of the source blocks to the interface required by the harnessed component. Modifying the contents of this subsystem may result in compilation and simulation failure.
  Inport_1 : Inport
  Inport_2 : Inport  Port=2
  Inport_3 : Inport  Port=3
  Inport_4 : Inport  Port=4
  Inport_5 : Inport  Port=5
  Inport_6 : Inport  Port=6
  Inport_7 : Inport  Port=7
  Inport_8 : Inport  Port=8
  Inport_9 : Inport  Port=9
  Inport_10 : Inport  Port=10
  Inport_11 : Inport  Port=11
  Inport_12 : Inport  Port=12
  Inport_13 : Inport  Port=13
  Inport_14 : Inport  Port=14
  Inport_15 : Inport  Port=15
  Inport_16 : Inport  Port=16
  Inport_17 : Inport  Port=17
  Inport_18 : Inport  Port=18
  Inport_19 : Inport  Port=19
  Inport_20 : Inport  Port=20
  Inport_21 : Inport  Port=21
  Inport_22 : Inport  Port=22
  Inport_23 : Inport  Port=23
  Inport_24 : Inport  Port=24
  Inport_25 : Inport  Port=25
  Inport_26 : Inport  Port=26
  Inport_27 : Inport  Port=27
  Inport_28 : Inport  Port=28
  Inport_29 : Inport  Port=29
  Inport_30 : Inport  Port=30
  Inport_31 : Inport  Port=31
  Inport_32 : Inport  Port=32
  Inport_33 : Inport  Port=33
  Inport_34 : Inport  Port=34
  Inport_35 : Inport  Port=35
  Inport_36 : Inport  Port=36
  Inport_37 : Inport  Port=37
  Inport_38 : Inport  Port=38
  Inport_39 : Inport  Port=39
  Inport_40 : Inport  Port=40
  Inport_41 : Inport  Port=41
  Inport_42 : Inport  Port=42
  Inport_43 : Inport  Port=43
  Inport_44 : Inport  Port=44
  Inport_45 : Inport  Port=45
  Inport_46 : Inport  Port=46
  Inport_47 : Inport  Port=47
  Inport_48 : Inport  Port=48
  Inport_49 : Inport  Port=49
  Data_Conversion_{1,3,13,16..18,21,24..31,34..37} (19 alike) : DataTypeConversion  OutDataTypeStr=boolean
  Data_Conversion_{6,10,12,14..15,19..20,33,38..46,49} (18 alike) : DataTypeConversion  OutDataTypeStr=uint8
  Data_Conversion_{2,4..5,7,9,11,32} (7 alike) : DataTypeConversion  OutDataTypeStr=single
  Data_Conversion_{8,22..23,47..48} (5 alike) : DataTypeConversion  OutDataTypeStr=uint16
  RateTs_{1..49} (49 alike) : RateTransition  OutPortSampleTime=0.01
  SigSpec_{1,3,13,16..18,21,24..31,34..37} (19 alike) : SignalSpecification  OutDataTypeStr=boolean  Unit=flag  Dimensions=[1]  SampleTime=0.01
  SigSpec_{6,10,12,38..45} (11 alike) : SignalSpecification  OutDataTypeStr=uint8  Unit=numb  Dimensions=[1]  SampleTime=0.01
  SigSpec_11 : SignalSpecification  OutDataTypeStr=single  Unit=C  Dimensions=[1]  SampleTime=0.01
  SigSpec_{14..15,19..20,33,46,49} (7 alike) : SignalSpecification  OutDataTypeStr=uint8  Unit=enum  Dimensions=[1]  SampleTime=0.01
  SigSpec_2 : SignalSpecification  OutDataTypeStr=single  Unit=V  Dimensions=[1]  SampleTime=0.01
  SigSpec_22 : SignalSpecification  OutDataTypeStr=uint16  Unit=mV  Dimensions=[1]  SampleTime=0.01
  SigSpec_23 : SignalSpecification  OutDataTypeStr=uint16  Unit=mV  Dimensions=[1]  SampleTime=0.01
  SigSpec_32 : SignalSpecification  OutDataTypeStr=single  Unit=V  Dimensions=[1]  SampleTime=0.01
  SigSpec_4 : SignalSpecification  OutDataTypeStr=single  Unit=A  Dimensions=[1]  SampleTime=0.01
  SigSpec_47 : SignalSpecification  OutDataTypeStr=uint16  Unit=mV  Dimensions=[1]  SampleTime=0.01
  SigSpec_48 : SignalSpecification  OutDataTypeStr=uint16  Unit=kWh  Dimensions=[1]  SampleTime=0.01
  SigSpec_5 : SignalSpecification  OutDataTypeStr=single  Unit=A  Dimensions=[1]  SampleTime=0.01
  SigSpec_7 : SignalSpecification  OutDataTypeStr=single  Unit=pct  Dimensions=[1]  SampleTime=0.01
  SigSpec_8 : SignalSpecification  OutDataTypeStr=uint16  Unit=min  Dimensions=[1]  SampleTime=0.01
  SigSpec_9 : SignalSpecification  OutDataTypeStr=single  Unit=C  Dimensions=[1]  SampleTime=0.01
  Outport_1 : Outport
  Outport_2 : Outport  Port=2
  Outport_3 : Outport  Port=3
  Outport_4 : Outport  Port=4
  Outport_5 : Outport  Port=5
  Outport_6 : Outport  Port=6
  Outport_7 : Outport  Port=7
  Outport_8 : Outport  Port=8
  Outport_9 : Outport  Port=9
  Outport_10 : Outport  Port=10
  Outport_11 : Outport  Port=11
  Outport_12 : Outport  Port=12
  Outport_13 : Outport  Port=13
  Outport_14 : Outport  Port=14
  Outport_15 : Outport  Port=15
  Outport_16 : Outport  Port=16
  Outport_17 : Outport  Port=17
  Outport_18 : Outport  Port=18
  Outport_19 : Outport  Port=19
  Outport_20 : Outport  Port=20
  Outport_21 : Outport  Port=21
  Outport_22 : Outport  Port=22
  Outport_23 : Outport  Port=23
  Outport_24 : Outport  Port=24
  Outport_25 : Outport  Port=25
  Outport_26 : Outport  Port=26
  Outport_27 : Outport  Port=27
  Outport_28 : Outport  Port=28
  Outport_29 : Outport  Port=29
  Outport_30 : Outport  Port=30
  Outport_31 : Outport  Port=31
  Outport_32 : Outport  Port=32
  Outport_33 : Outport  Port=33
  Outport_34 : Outport  Port=34
  Outport_35 : Outport  Port=35
  Outport_36 : Outport  Port=36
  Outport_37 : Outport  Port=37
  Outport_38 : Outport  Port=38
  Outport_39 : Outport  Port=39
  Outport_40 : Outport  Port=40
  Outport_41 : Outport  Port=41
  Outport_42 : Outport  Port=42
  Outport_43 : Outport  Port=43
  Outport_44 : Outport  Port=44
  Outport_45 : Outport  Port=45
  Outport_46 : Outport  Port=46
  Outport_47 : Outport  Port=47
  Outport_48 : Outport  Port=48
  Outport_49 : Outport  Port=49
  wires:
  SigSpec_1/1 -> Outport_1/1
  RateTs_1/1 -> SigSpec_1/1
  Data_Conversion_1/1 -> RateTs_1/1
  Inport_1/1 -> Data_Conversion_1/1
  SigSpec_2/1 -> Outport_2/1
  RateTs_2/1 -> SigSpec_2/1
  Data_Conversion_2/1 -> RateTs_2/1
  Inport_2/1 -> Data_Conversion_2/1
  SigSpec_3/1 -> Outport_3/1
  RateTs_3/1 -> SigSpec_3/1
  Data_Conversion_3/1 -> RateTs_3/1
  Inport_3/1 -> Data_Conversion_3/1
  SigSpec_4/1 -> Outport_4/1
  RateTs_4/1 -> SigSpec_4/1
  Data_Conversion_4/1 -> RateTs_4/1
  Inport_4/1 -> Data_Conversion_4/1
  SigSpec_5/1 -> Outport_5/1
  RateTs_5/1 -> SigSpec_5/1
  Data_Conversion_5/1 -> RateTs_5/1
  Inport_5/1 -> Data_Conversion_5/1
  SigSpec_6/1 -> Outport_6/1
  RateTs_6/1 -> SigSpec_6/1
  Data_Conversion_6/1 -> RateTs_6/1
  Inport_6/1 -> Data_Conversion_6/1
  SigSpec_7/1 -> Outport_7/1
  RateTs_7/1 -> SigSpec_7/1
  Data_Conversion_7/1 -> RateTs_7/1
  Inport_7/1 -> Data_Conversion_7/1
  SigSpec_8/1 -> Outport_8/1
  RateTs_8/1 -> SigSpec_8/1
  Data_Conversion_8/1 -> RateTs_8/1
  Inport_8/1 -> Data_Conversion_8/1
  SigSpec_9/1 -> Outport_9/1
  RateTs_9/1 -> SigSpec_9/1
  Data_Conversion_9/1 -> RateTs_9/1
  Inport_9/1 -> Data_Conversion_9/1
  SigSpec_10/1 -> Outport_10/1
  RateTs_10/1 -> SigSpec_10/1
  Data_Conversion_10/1 -> RateTs_10/1
  Inport_10/1 -> Data_Conversion_10/1
  SigSpec_11/1 -> Outport_11/1
  RateTs_11/1 -> SigSpec_11/1
  Data_Conversion_11/1 -> RateTs_11/1
  Inport_11/1 -> Data_Conversion_11/1
  SigSpec_12/1 -> Outport_12/1
  RateTs_12/1 -> SigSpec_12/1
  Data_Conversion_12/1 -> RateTs_12/1
  Inport_12/1 -> Data_Conversion_12/1
  SigSpec_13/1 -> Outport_13/1
  RateTs_13/1 -> SigSpec_13/1
  Data_Conversion_13/1 -> RateTs_13/1
  Inport_13/1 -> Data_Conversion_13/1
  SigSpec_14/1 -> Outport_14/1
  RateTs_14/1 -> SigSpec_14/1
  Data_Conversion_14/1 -> RateTs_14/1
  Inport_14/1 -> Data_Conversion_14/1
  SigSpec_15/1 -> Outport_15/1
  RateTs_15/1 -> SigSpec_15/1
  Data_Conversion_15/1 -> RateTs_15/1
  Inport_15/1 -> Data_Conversion_15/1
  SigSpec_16/1 -> Outport_16/1
  RateTs_16/1 -> SigSpec_16/1
  Data_Conversion_16/1 -> RateTs_16/1
  Inport_16/1 -> Data_Conversion_16/1
  SigSpec_17/1 -> Outport_17/1
  RateTs_17/1 -> SigSpec_17/1
  Data_Conversion_17/1 -> RateTs_17/1
  Inport_17/1 -> Data_Conversion_17/1
  SigSpec_18/1 -> Outport_18/1
  RateTs_18/1 -> SigSpec_18/1
  Data_Conversion_18/1 -> RateTs_18/1
  Inport_18/1 -> Data_Conversion_18/1
  SigSpec_19/1 -> Outport_19/1
  RateTs_19/1 -> SigSpec_19/1
  Data_Conversion_19/1 -> RateTs_19/1
  Inport_19/1 -> Data_Conversion_19/1
  SigSpec_20/1 -> Outport_20/1
  RateTs_20/1 -> SigSpec_20/1
  Data_Conversion_20/1 -> RateTs_20/1
  Inport_20/1 -> Data_Conversion_20/1
  SigSpec_21/1 -> Outport_21/1
  RateTs_21/1 -> SigSpec_21/1
  Data_Conversion_21/1 -> RateTs_21/1
  Inport_21/1 -> Data_Conversion_21/1
  SigSpec_22/1 -> Outport_22/1
  RateTs_22/1 -> SigSpec_22/1
  Data_Conversion_22/1 -> RateTs_22/1
  Inport_22/1 -> Data_Conversion_22/1
  SigSpec_23/1 -> Outport_23/1
  RateTs_23/1 -> SigSpec_23/1
  Data_Conversion_23/1 -> RateTs_23/1
  Inport_23/1 -> Data_Conversion_23/1
  SigSpec_24/1 -> Outport_24/1
  RateTs_24/1 -> SigSpec_24/1
  Data_Conversion_24/1 -> RateTs_24/1
  Inport_24/1 -> Data_Conversion_24/1
  SigSpec_25/1 -> Outport_25/1
  RateTs_25/1 -> SigSpec_25/1
  Data_Conversion_25/1 -> RateTs_25/1
  Inport_25/1 -> Data_Conversion_25/1
  SigSpec_26/1 -> Outport_26/1
  RateTs_26/1 -> SigSpec_26/1
  Data_Conversion_26/1 -> RateTs_26/1
  Inport_26/1 -> Data_Conversion_26/1
  SigSpec_27/1 -> Outport_27/1
  RateTs_27/1 -> SigSpec_27/1
  Data_Conversion_27/1 -> RateTs_27/1
  Inport_27/1 -> Data_Conversion_27/1
  SigSpec_28/1 -> Outport_28/1
  RateTs_28/1 -> SigSpec_28/1
  Data_Conversion_28/1 -> RateTs_28/1
  Inport_28/1 -> Data_Conversion_28/1
  SigSpec_29/1 -> Outport_29/1
  RateTs_29/1 -> SigSpec_29/1
  Data_Conversion_29/1 -> RateTs_29/1
  Inport_29/1 -> Data_Conversion_29/1
  SigSpec_30/1 -> Outport_30/1
  RateTs_30/1 -> SigSpec_30/1
  Data_Conversion_30/1 -> RateTs_30/1
  Inport_30/1 -> Data_Conversion_30/1
  SigSpec_31/1 -> Outport_31/1
  RateTs_31/1 -> SigSpec_31/1
  Data_Conversion_31/1 -> RateTs_31/1
  Inport_31/1 -> Data_Conversion_31/1
  SigSpec_32/1 -> Outport_32/1
  RateTs_32/1 -> SigSpec_32/1
  Data_Conversion_32/1 -> RateTs_32/1
  Inport_32/1 -> Data_Conversion_32/1
  SigSpec_33/1 -> Outport_33/1
  RateTs_33/1 -> SigSpec_33/1
  Data_Conversion_33/1 -> RateTs_33/1
  Inport_33/1 -> Data_Conversion_33/1
  SigSpec_34/1 -> Outport_34/1
  RateTs_34/1 -> SigSpec_34/1
  Data_Conversion_34/1 -> RateTs_34/1
  Inport_34/1 -> Data_Conversion_34/1
  SigSpec_35/1 -> Outport_35/1
  RateTs_35/1 -> SigSpec_35/1
  Data_Conversion_35/1 -> RateTs_35/1
  Inport_35/1 -> Data_Conversion_35/1
  SigSpec_36/1 -> Outport_36/1
  RateTs_36/1 -> SigSpec_36/1
  Data_Conversion_36/1 -> RateTs_36/1
  Inport_36/1 -> Data_Conversion_36/1
  SigSpec_37/1 -> Outport_37/1
  RateTs_37/1 -> SigSpec_37/1
  Data_Conversion_37/1 -> RateTs_37/1
  Inport_37/1 -> Data_Conversion_37/1
  SigSpec_38/1 -> Outport_38/1
  RateTs_38/1 -> SigSpec_38/1
  Data_Conversion_38/1 -> RateTs_38/1
  Inport_38/1 -> Data_Conversion_38/1
  SigSpec_39/1 -> Outport_39/1
  RateTs_39/1 -> SigSpec_39/1
  Data_Conversion_39/1 -> RateTs_39/1
  Inport_39/1 -> Data_Conversion_39/1
  SigSpec_40/1 -> Outport_40/1
  RateTs_40/1 -> SigSpec_40/1
  Data_Conversion_40/1 -> RateTs_40/1
  Inport_40/1 -> Data_Conversion_40/1
  SigSpec_41/1 -> Outport_41/1
  RateTs_41/1 -> SigSpec_41/1
  Data_Conversion_41/1 -> RateTs_41/1
  Inport_41/1 -> Data_Conversion_41/1
  SigSpec_42/1 -> Outport_42/1
  RateTs_42/1 -> SigSpec_42/1
  Data_Conversion_42/1 -> RateTs_42/1
  Inport_42/1 -> Data_Conversion_42/1
  SigSpec_43/1 -> Outport_43/1
  RateTs_43/1 -> SigSpec_43/1
  Data_Conversion_43/1 -> RateTs_43/1
  Inport_43/1 -> Data_Conversion_43/1
  SigSpec_44/1 -> Outport_44/1
  RateTs_44/1 -> SigSpec_44/1
  Data_Conversion_44/1 -> RateTs_44/1
  Inport_44/1 -> Data_Conversion_44/1
  SigSpec_45/1 -> Outport_45/1
  RateTs_45/1 -> SigSpec_45/1
  Data_Conversion_45/1 -> RateTs_45/1
  Inport_45/1 -> Data_Conversion_45/1
  SigSpec_46/1 -> Outport_46/1
  RateTs_46/1 -> SigSpec_46/1
  Data_Conversion_46/1 -> RateTs_46/1
  Inport_46/1 -> Data_Conversion_46/1
  SigSpec_47/1 -> Outport_47/1
  RateTs_47/1 -> SigSpec_47/1
  Data_Conversion_47/1 -> RateTs_47/1
  Inport_47/1 -> Data_Conversion_47/1
  SigSpec_48/1 -> Outport_48/1
  RateTs_48/1 -> SigSpec_48/1
  Data_Conversion_48/1 -> RateTs_48/1
  Inport_48/1 -> Data_Conversion_48/1
  SigSpec_49/1 -> Outport_49/1
  RateTs_49/1 -> SigSpec_49/1
  Data_Conversion_49/1 -> RateTs_49/1
  Inport_49/1 -> Data_Conversion_49/1
